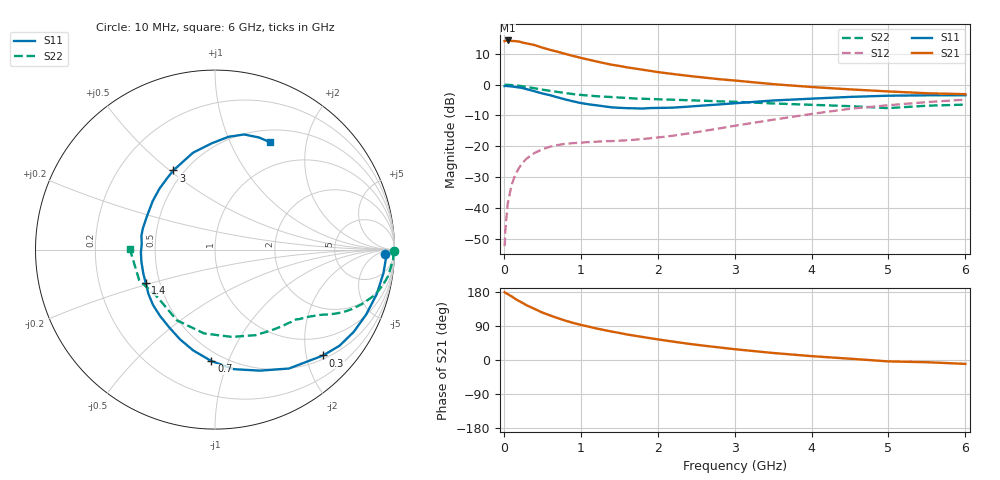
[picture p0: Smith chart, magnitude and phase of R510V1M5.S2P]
! SIEMENS Small Signal Semiconductors
! BFR183
! Si NPN RF Bipolar Junction Transistor in SOT23
! VCE = 10 V  IC = 1.5 mA
! Common Emitter S-Parameters:  May  1996
# GHz  S  MA  R  50
!  f  S11  S21  S12  S22
! GHz  MAG  ANG  MAG  ANG  MAG  ANG  MAG  ANG
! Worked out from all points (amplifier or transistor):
!   36 points, 10 MHz to 6 GHz, reference 50 ohm
!   highest |S21| = 14.3 dB at 50 MHz (marker M1)
!   |S21| within 3 dB of that: start of sweep to 594.3 MHz
!   unconditionally stable (mu >= 1): 1.551 GHz to 2.923 GHz
!   at 250 MHz: K = 0.19, MSG = 19.4 dB, |S12| = -25.2 dB
!   at 1.4 GHz: K = 0.93, MSG = 12.4 dB, |S12| = -18.3 dB
!   at 6 GHz: K = 0.91, MSG = 0.9 dB, |S12| = -4.9 dB
!   S11 on the Smith chart (normalised r, x): 10 MHz: 30, -16; 300 MHz: 0.57, -2.33; 700 MHz: 0.43, -0.87; 1.4 GHz: 0.42, -0.19; 3 GHz: 0.44, +0.51; 6 GHz: 0.65, +1.43
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0.01  0.9489 -1.6  5.093 179.0  0.0024 91.4  0.9952 -0.6
0.02  0.9534 -3.1  5.129 177.3  0.0044 85.3  0.9943 -1.2
0.05  0.9474 -8.0  5.208 173.9  0.0117 84.2  0.9941 -3.1
0.1  0.9346 -15.4  5.114 168.1  0.0234 81.1  0.9837 -6.0
0.15  0.9165 -23.3  5.079 161.1  0.0349 76.6  0.9744 -8.9
0.2  0.8986 -30.7  4.985 155.4  0.045 71.9  0.9577 -11.6
0.3  0.843 -44.4  4.656 144.1  0.0639 64.8  0.9205 -16.3
0.4  0.7803 -58.1  4.382 134.7  0.078 58.4  0.8735 -20.3
0.5  0.7196 -69.6  3.98 125.3  0.0894 53.1  0.83 -23.6
0.6  0.6743 -81.1  3.67 117.7  0.0985 48.7  0.7947 -26.0
0.7  0.6216 -91.8  3.414 110.5  0.1051 45.5  0.7613 -27.9
0.8  0.5747 -102.2  3.149 103.9  0.1096 42.5  0.7311 -29.6
0.9  0.5363 -111.4  2.924 97.9  0.1126 41.0  0.7019 -31.1
1.1  0.4805 -129.5  2.546 88.2  0.117 39.3  0.6651 -33.7
1.4  0.4281 -154.5  2.107 75.1  0.1215 39.0  0.6295 -37.2
1.7  0.4131 -177.7  1.83 64.1  0.1278 42.8  0.5961 -40.7
2.2  0.4237 152.2  1.487 48.5  0.1485 49.8  0.5692 -48.1
3  0.4985 117.8  1.167 28.5  0.2152 55.1  0.5274 -64.7
3.5  0.5531 102.9  1.019 18.5  0.2698 53.0  0.4952 -79.1
4.5  0.6329 83.2  0.838 3.4  0.406 42.2  0.4475 -118.4
5.5  0.671 68.6  0.725 -5.8  0.5215 27.0  0.4556 -157.9
6  0.6722 62.9  0.701 -10.3  0.5707 17.6  0.4743 179.7
